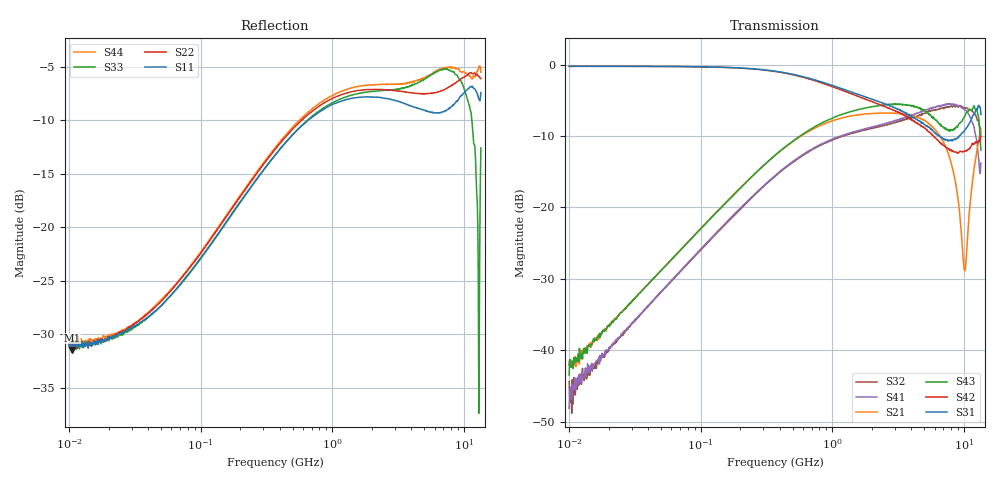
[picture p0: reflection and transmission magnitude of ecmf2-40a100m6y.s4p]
!ECMF2-40A100M6Y
!Typical device
!Port 1: IN1
!Port 2: IN2
!Port 3: OUT1
!Port 4: OUT2
!Start Freq. :100.000MHz; Stop Freq. : 13.500GHz
!Number of points : 801; Sweep : LOGARITHMIC
!Ports power : -5.000000dBm; IFBW : 100.000000Hz
# Hz S  RI  R 50
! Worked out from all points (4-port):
!   801 points, 10 MHz to 13.5 GHz, reference 50 ohm
!   strongest paths, dB at 10 MHz, 60.62 MHz, 367.4 MHz, 2.227 GHz, 13.5 GHz:
!     S31: -0.2, -0.3, -0.9, -5.1, -7.0
!     S42: -0.2, -0.3, -1.0, -5.5, -10.1
!     S43: -43.5, -27.3, -12.7, -5.8, -12.0
!     S21: -42.1, -27.2, -12.7, -6.8, -9.0
!     S41: -48.1, -30.2, -15.6, -8.5, -13.8
!     S32: -44.4, -30.3, -15.6, -8.7, -9.9
!   lowest |S11| = -31.5 dB at 10.46 MHz (marker M1), VSWR 1.05, Z = 52.6 + j0.742 ohm
!   |S11| at or under -10 dB: start of sweep to 654.1 MHz
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1e7  0.0282 0.00571  0.00195 0.00788  0.9728 -0.0134  -0.000881 -0.00579
     0.000443 0.00789  0.0276 0.00228  -0.00118 -0.00466  0.9725 -0.0116
     0.9723 -0.0123  -0.000684 -0.00599  0.0278 0.00644  0.000657 0.00781
     -0.000498 -0.00388  0.9724 -0.0125  0.000204 0.00666  0.0274 0.00741
1.046079e7  0.0257 0.00704  0.00128 0.00764  0.9728 -0.0126  -0.000732 -0.0054
            -0.000104 0.00762  0.0291 0.00589  0.000133 -0.0051  0.9721 -0.0112
            0.9712 -0.011  -8.81e-05 -0.00361  0.028 0.00499  0.00165 0.00885
            0.000466 -0.00452  0.9705 -0.0106  0.000419 0.00765  0.0272 0.00647
3.480883e8  0.1339 0.1593  0.1139 0.1897  0.8563 -0.2932  -0.0993 -0.1251
            0.114 0.1897  0.1416 0.1705  -0.0971 -0.1246  0.8456 -0.3083
            0.8561 -0.2931  -0.097 -0.1247  0.1225 0.1684  0.1044 0.1957
            -0.0993 -0.1253  0.8473 -0.3077  0.1043 0.1958  0.1333 0.182
4.036481e9  0.1541 -0.334  0.3518 -0.2607  -0.1454 -0.4105  0.174 0.4087
            0.3524 -0.2604  0.1867 -0.382  0.1448 0.4031  -0.1604 -0.38
            -0.1433 -0.4094  0.1432 0.4018  0.4295 -0.1636  0.4668 -0.2153
            0.171 0.4084  -0.158 -0.3793  0.4677 -0.2143  0.4274 -0.2099
7.584153e9  -0.324 -0.1471  -0.0314 -0.2369  -0.2129 0.1928  0.4702 -0.2131
            -0.0313 -0.2404  -0.3495 -0.2824  0.4761 -0.1633  -0.1943 0.1629
            -0.2234 0.1859  0.481 -0.1442  0.1461 -0.526  0.2138 -0.2707
            0.4922 -0.2004  -0.203 0.1581  0.2166 -0.276  0.1469 -0.5405
1.01186e10  -0.2571 0.3396  -0.0293 0.0195  0.1808 0.2732  0.0412 -0.4504
            -0.0297 0.0204  -0.4694 0.1871  0.12 -0.4672  0.1159 0.2052
            0.1865 0.2896  0.1376 -0.4778  -0.2746 -0.3427  0.1709 -0.3889
            0.0467 -0.4796  0.116 0.2168  0.1707 -0.395  -0.2478 -0.47
1.35e10  0.2725 0.3284  0.34 -0.108  0.2855 -0.3107  -0.1253 -0.1474
         0.3368 -0.1059  0.0916 0.4868  -0.2912 -0.0689  0.2927 0.0103
         0.3068 -0.3255  -0.3112 -0.0768  0.0433 -0.2311  -0.1273 -0.2179
         -0.1422 -0.1467  0.3123 -0.00991  -0.1431 -0.2066  -0.5203 0.1068
